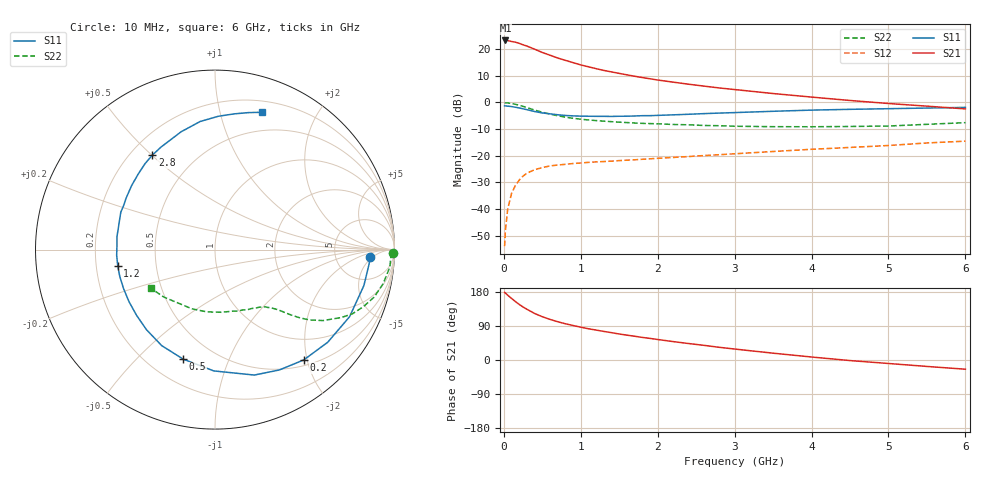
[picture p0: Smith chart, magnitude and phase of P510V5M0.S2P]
! SIEMENS Small Signal Semiconductors
! BFP183
! Si NPN RF Bipolar Junction Transistor in SOT143
! VCE = 10 V  IC = 5 mA
! Common Emitter S-Parameters:  March  1996
# GHz  S  MA  R  50
!  f  S11  S21  S12  S22
! GHz  MAG  ANG  MAG  ANG  MAG  ANG  MAG  ANG
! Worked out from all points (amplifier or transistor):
!   36 points, 10 MHz to 6 GHz, reference 50 ohm
!   highest |S21| = 23.3 dB at 20 MHz (marker M1)
!   |S21| within 3 dB of that: start of sweep to 376.5 MHz
!   unconditionally stable (mu >= 1): 1.666 GHz to 5.777 GHz
!   at 250 MHz: K = 0.20, MSG = 24.7 dB, |S12| = -27.7 dB
!   at 1.4 GHz: K = 0.90, MSG = 16.7 dB, |S12| = -22.0 dB
!   at 6 GHz: K = 0.97, MSG = 6.1 dB, |S12| = -14.5 dB
!   S11 on the Smith chart (normalised r, x): 10 MHz: 13, -4; 200 MHz: 0.60, -1.94; 500 MHz: 0.34, -0.69; 1.2 GHz: 0.29, -0.07; 2.8 GHz: 0.29, +0.50; 6 GHz: 0.31, +1.35
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0.01  0.865 -2.6  14.55 178.1  0.002 78.0  0.9898 -1.1
0.02  0.862 -5.5  14.61 176.6  0.0039 83.1  0.9805 -2.3
0.05  0.8534 -13.6  14.56 171.0  0.0099 83.5  0.9791 -5.7
0.15  0.813 -39.4  13.57 154.2  0.0276 68.7  0.9256 -16.6
0.2  0.7889 -51.2  12.91 146.7  0.0348 63.8  0.885 -21.1
0.25  0.7602 -61.9  12.09 139.9  0.0414 58.8  0.8456 -25.0
0.3  0.7325 -72.6  11.46 133.9  0.047 54.0  0.8001 -28.2
0.4  0.6759 -90.6  10.02 122.8  0.0545 47.5  0.7201 -33.3
0.5  0.6355 -106.2  8.677 114.2  0.0599 42.0  0.6556 -36.7
0.6  0.6119 -119.0  7.726 107.2  0.0643 38.7  0.6042 -38.9
0.7  0.5875 -130.4  6.832 101.0  0.0668 35.7  0.5629 -40.5
0.8  0.5703 -140.0  6.185 95.6  0.069 33.6  0.5304 -41.8
1.1  0.5513 -164.2  4.681 82.4  0.075 30.8  0.4692 -44.7
1.2  0.5492 -170.7  4.313 79.0  0.0765 29.9  0.4571 -45.6
1.5  0.551 172.5  3.517 68.6  0.0809 29.6  0.4264 -48.5
1.7  0.557 162.6  3.109 62.7  0.0838 29.9  0.4113 -51.2
2.2  0.5857 142.5  2.41 48.6  0.0927 30.1  0.3862 -58.2
2.8  0.6317 123.5  1.874 33.5  0.1044 29.7  0.3661 -69.1
3.5  0.6829 106.1  1.472 18.0  0.12 28.8  0.3509 -84.3
4.5  0.743 88.6  1.09 -1.5  0.143 25.2  0.3541 -111.2
5.5  0.7856 76.3  0.853 -17.0  0.1737 21.0  0.3886 -137.0
6  0.8086 71.1  0.757 -24.3  0.1876 17.5  0.4177 -149.0
